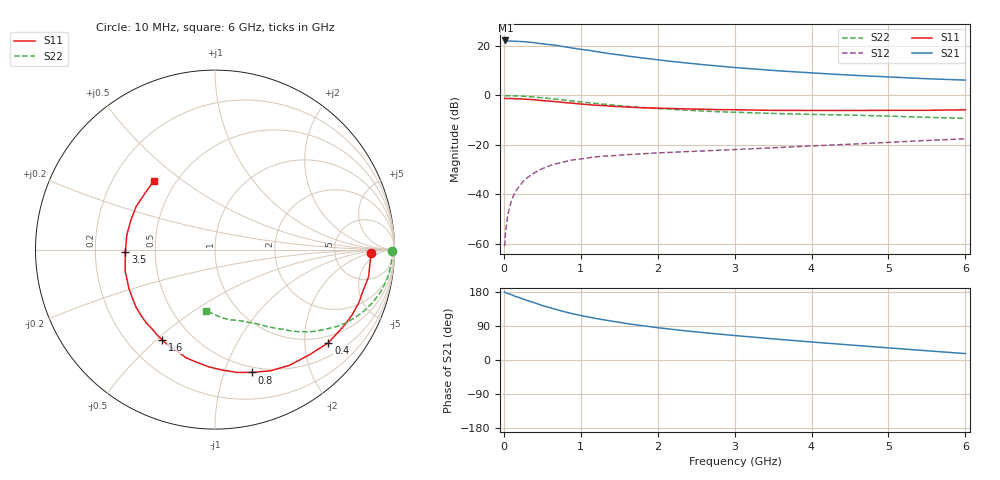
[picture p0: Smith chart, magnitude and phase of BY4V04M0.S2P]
! SIEMENS Small Signal Semiconductors
! BFY420
! Si NPN RF SIEGET Grounded Emitter Transistor in MICRO-X
! VCE = 4 V  IC = 4 mA
! Common Emitter S-Parameters:  October  1996
# GHz  S  MA  R  50
!  f  S11  S21  S12  S22
! GHz  MAG  ANG  MAG  ANG  MAG  ANG  MAG  ANG
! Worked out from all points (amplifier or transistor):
!   36 points, 10 MHz to 6 GHz, reference 50 ohm
!   highest |S21| = 22.2 dB at 20 MHz (marker M1)
!   |S21| within 3 dB of that: start of sweep to 877.3 MHz
!   unconditionally stable (mu >= 1): 3.348 GHz to end of sweep
!   at 250 MHz: K = 0.13, MSG = 28.3 dB, |S12| = -34.8 dB
!   at 1.4 GHz: K = 0.46, MSG = 20.6 dB, |S12| = -24.4 dB
!   at 6 GHz: K = 1.15, MAG = 9.5 dB, |S12| = -17.5 dB
!   S11 on the Smith chart (normalised r, x): 10 MHz: 14, -2; 400 MHz: 0.82, -2.56; 800 MHz: 0.45, -1.25; 1.6 GHz: 0.34, -0.52; 3.5 GHz: 0.33, -0.01; 6 GHz: 0.38, +0.39
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0.01  0.8691 -1.3  12.91 179.7  0.0009 33.0  0.9888 -0.5
0.02  0.869 -2.2  12.93 177.7  0.0016 55.3  0.9857 -0.9
0.05  0.8671 -5.1  12.57 175.4  0.0038 72.2  0.9878 -2.3
0.1  0.869 -10.1  12.54 172.5  0.0077 80.6  0.9838 -4.8
0.15  0.8566 -15.2  12.43 167.7  0.0114 77.0  0.9786 -7.3
0.3  0.8366 -30.0  12.05 157.2  0.0216 73.0  0.9537 -14.1
0.4  0.8177 -39.4  11.62 151.0  0.0275 67.8  0.9272 -18.5
0.5  0.7863 -48.5  11.07 143.6  0.0332 64.2  0.898 -22.4
0.6  0.7663 -57.4  10.65 138.0  0.0383 60.3  0.8666 -26.0
0.7  0.7429 -65.3  10.15 132.2  0.0425 56.7  0.8339 -29.4
0.8  0.7147 -73.2  9.57 126.8  0.0462 53.2  0.8006 -32.4
0.9  0.6951 -79.9  9.032 121.8  0.0499 50.6  0.7706 -34.8
1.1  0.6537 -93.2  8.173 113.5  0.055 46.3  0.7149 -39.6
1.3  0.6245 -104.8  7.305 106.0  0.0594 42.8  0.6655 -43.3
1.6  0.5837 -120.2  6.277 96.1  0.0637 39.3  0.6037 -48.1
1.8  0.5629 -128.9  5.721 90.5  0.0661 37.6  0.572 -50.6
2.2  0.5443 -144.0  4.832 80.6  0.0713 35.4  0.5233 -55.4
2.8  0.5171 -161.5  3.92 68.3  0.0783 33.8  0.4688 -61.4
3.5  0.4999 -178.6  3.202 55.8  0.0876 32.7  0.4325 -67.7
4.5  0.4966 160.5  2.574 39.7  0.1035 30.3  0.4011 -77.6
5.5  0.5008 140.8  2.177 24.4  0.1232 26.5  0.3617 -90.3
6  0.5126 131.8  2.043 16.9  0.1332 23.9  0.3449 -97.9
